PROGRAM MAIN
VAR
	bInitialized 		: 	BOOL := FALSE;
	bDeinitialize		:	BOOL;
	bCheck				:	BOOL;
	fbInit 				: 	FB_VN_InitializeFunction;	
	nReturnCode			:   UDINT;
	
	hr					:	HRESULT;
	hrCheck				:	HRESULT;
	hrDeinitialize		:	HRESULT;
	hrOCR				:	HRESULT;
	fbCameraControl		:	FB_VN_FileSourceControl;
	eCameraState		:	ETcVnCameraState;
	sFileName 			: 	STRING;
	ImageCounter		:	UINT;

	stPixelFormat		:	TcVnPixelFormat;
	stRoi				:	TcVnRectangle_UDINT;
	fThreshold			:	LREAL;
	bInvertImage		:	BOOL := TRUE;
	
	ipOriginalImage		:	ITcVnImage; 
	ipBinaryImage		:	ITcVnImage; 
	ipThreshBorder		:	ITcVnImage;
	ipStructElem		: 	ITcvnImage;
	ipOriginImageDisp	:	ITcVnDisplayableImage;
	ipBinImageDisp		:	ITcVnDisplayableImage;
	ipThreshBorderDisp	:	ITcVnDisplayableImage;
	
	aRedColor			: 	TcVnVector4_LREAL := [255,0,0];
	aGreenColor			: 	TcVnVector4_LREAL := [0,255,0];
	aBlueColor			: 	TcVnVector4_LREAL := [0,0,255];
	aWhiteColor			: 	TcVnVector4_LREAL := [255,255,255];
	
	// OCR
	bUseExpFunction		:	BOOL := FALSE;
	ipOCRResult 		:	ITcVnContainer; (* Returns the detected characters (ContainerType_Vector_String_SINT) *)
	sText 				: 	STRING(255);
	nStringLenght		:	INT;

	// OCR Exp
	sPattern			:	STRING;			(* String template containing the format in which characters are presented *)
	eOcrOptions			:	UDINT;			(* Specifies which options must be applied to the function (ETcVnOcrOptions) *)
	ipBoundingBoxes		:	ITcVnContainer;	(* Returns the corresponding bounding boxes of the detected characters (ContainerType_Vector_TcVnRectangle_DINT, optional, set to 0 if not required) *)
	ipConfidences		:	ITcVnContainer;	(* Returns the corresponding classification confidences of the detected characters (ContainerType_Vector_REAL, optional, set to 0 if not required) *)
	fMinConfidence		:	REAL;			(* Returns the minimum value of the confidences *)
	
	nNumberOfElements	: 	ULINT;
	nIterator			: 	ULINT;
	aConfidences		:	ARRAY [0..11] OF REAL;
	stRectangle			:	TcVnRectangle_DINT;
END_VAR

// Disclaimer

// This publication contains statements about the suitability of our products for certain
// areas of application. These statements are based on typical features of our products.
// The examples shown in this publication are for demonstration purposes only.
// The information provided herein should not be regarded as specific operation characteristics.
// It is incumbent on the customer to check and decide whether a product is suitable for use
// in a particular application. We do not give any warranty that the source code which is
// made available with this publication is complete or accurate.

// THE SAMPLE CODE CONTAINED IN THIS PUBLICATION IS PROVIDED “AS IS” WITHOUT WARRANTY OF ANY KIND,
// EITHER EXPRESSED, IMPLIED OR STATUTORY, INCLUDING WITHOUT LIMITATION, ANY WARRANTY WITH RESPECT TO NON-INFRINGEMENT,
// FREEDOM FROM PROPRIETARY RIGHTS OF THIRD PARTIES OR FITNESS FOR ANY PARTICULAR PURPOSE.

// This publication may be changed from time to time without prior notice.
// No liability is assumed for errors and/or omissions.
// Our products are described in detail in our data sheets and documentations.
// Product-specific warnings and cautions must be observed.
// For the latest version of our data sheets and documentations visit our website (www.beckhoff.de).

// © Beckhoff Automation GmbH & Co. KG, December 2023

// The reproduction, distribution and utilization of this document as well as the communication
// of its contents to others without express authorization is prohibited. 
// Offenders will be held liable for the payment of damages.
// All rights reserved in the event of the grant of a patent, utility model or design.

//	==========================================================================================

// SAMPLE - OCR (Optical Character Recognition)
//	-------------------------------------------------------

// Steps To Do:
// ------------
// 1. Add the sample images to the FileSource1 Control
// 2. Activate the Configuration -> Start TwinCAT System and PLC to run -> watch the results in the ADS Image Watch
// 3. Switch between OCR standard and expert function with bUseExpFunction

// Load OCR Model
IF NOT bInitialized THEN
	fbInit(eFunction := TCVN_IF_OCR, nOptions := ETcVnOcrModelType.TCVN_OMT_NUMBERS_SC_UCLETTERS OR ETcVnOcrModelType.TCVN_OMT_NUMBERS_SC OR ETcVnOcrModelType.TCVN_OMT_UCLETTERS, bStart := TRUE);
	
	IF NOT fbInit.bBusy THEN
		fbInit(bStart := FALSE);
		IF NOT fbInit.bError THEN
			bInitialized := TRUE;
			nReturnCode := fbInit.nErrorId AND 16#FFF;
		ELSE
			nReturnCode := fbInit.nErrorId AND 16#FFF;
		END_IF
	END_IF
END_IF

// Check if Model is initialized
IF bCheck THEN
	bCheck := FALSE;
	hrCheck := F_VN_CheckFunctionInitialization(eFunction := TCVN_IF_OCR, nOptions := ETcVnOcrModelType.TCVN_OMT_NUMBERS_SC, hrPrev := S_OK);
END_IF

// Unload OCR Model
IF bDeinitialize THEN
	bDeinitialize := FALSE;
	hrDeinitialize := F_VN_DeinitializeFunction(eFunction:= TCVN_IF_OCR, nOptions:= ETcVnOcrModelType.TCVN_OMT_NUMBERS_SC, hrPrev:= S_OK);
	bInitialized := FALSE;
END_IF

// Get Camera State
eCameraState := fbCameraControl.GetState();
	
// CameraControl is in error state, so try to reset the camera connection
IF eCameraState = TCVN_CS_ERROR THEN
	hr := fbCameraControl.Reset();

// Camera not yet streaming
ELSIF eCameraState < TCVN_CS_ACQUIRING THEN
	hr := fbCameraControl.StartAcquisition();

// Camera streaming
ELSIF eCameraState = TCVN_CS_ACQUIRING THEN	
	
	hr := fbCameraControl.GetCurrentImageAndFileName(ipImage := ipOriginalImage, sFileName := sFileName, 80);
	
	IF bInitialized AND SUCCEEDED(hr) AND ipOriginalImage <> 0 THEN
		
		ImageCounter := ImageCounter + 1;
		
		// Check pixel format and prepare work image
		hr := F_VN_GetPixelFormat(ipOriginalImage, stPixelFormat, hr);			
		IF stPixelFormat.nChannels = 3 AND stPixelFormat.ePixelEncoding = TCVN_PE_NONE THEN
			hr := F_VN_ConvertColorSpace(ipOriginalImage, ipBinaryImage, TCVN_CST_RGB_TO_GRAY, hr);			
		ELSE
			hr := F_VN_CopyImage(ipOriginalImage, ipBinaryImage, hr);
		END_IF
		
		// Helper funtion to get ROI and threshold value according to sample image
		F_GetROI(sFileName, stRoi, fThreshold, bInvertImage, sPattern);
			 
		// Set ROI and draw rectangle
		hr := F_VN_SetRoi_TcVnRectangle_UDINT(stRoi, ipBinaryImage, hr);
		hr := F_VN_DrawRectangle_TcVnRectangle_UDINT(stRoi, ipOriginalImage, aRedColor, 2, hr);
		
		// Filter Image 
		// Add or replace pre-processing functions if needed
		hr := F_VN_CreateStructuringElement(ipStructElem, ETcVnStructuringElementShape.TCVN_SES_RECTANGLE, 3,3, hr);
		hr := F_VN_MorphologicalOperator(ipBinaryImage, ipBinaryImage, ETcvnMorphologicalOperator.TCVN_MO_CLOSING_BY_RECONSTRUCTION, ipStructElem, hr);	

////		// Invert image depending on bright or dark text color 
		IF bInvertImage THEN
			hr := F_VN_Threshold(ipBinaryImage, ipBinaryImage, fThreshold, 255, TCVN_TT_BINARY_INV, hr);
		ELSE
			hr := F_VN_Threshold(ipBinaryImage, ipBinaryImage, fThreshold, 255, TCVN_TT_BINARY, hr);
		END_IF
		
		// Remove border objects
		hr := F_VN_BrightBorderObjects(ipBinaryImage, ipThreshBorder, hr);
		hr := F_VN_SubtractImages(ipBinaryImage, ipThreshBorder, ipBinaryImage, hr);
	
		// Read characters
		IF NOT bUseExpFunction THEN
			hrOCR := F_VN_OCR(
					ipSrcImage		:= ipBinaryImage,
					eModel			:= ETcVnOcrModelType.TCVN_OMT_NUMBERS_SC_UCLETTERS,
					ipCharacters	:= ipOCRResult,
					hrPrev			:= hr);
			hrOCR := F_VN_OCR(
					ipSrcImage		:= ipBinaryImage,
					eModel			:= ETcVnOcrModelType.TCVN_OMT_NUMBERS,
					ipCharacters	:= ipOCRResult,
					hrPrev			:= hr);
		ELSE
			hrOCR := F_VN_OCRExp(
					ipSrcImage		:= ipBinaryImage,
					eModel			:= ETcVnOcrModelType.TCVN_OMT_NUMBERS_SC or ETcVnOcrModelType.TCVN_OMT_UCLETTERS,
					ipCharacters	:= ipOCRResult, 
					sPattern		:= sPattern,
					eOcrOptions		:= eOcrOptions,
					ipBoundingBoxes	:= ipBoundingBoxes, 
					ipConfidences	:= ipConfidences,
					hrPrev			:= hr,
					fMinConfidence	=> fMinConfidence);
		END_IF
				
		// Check if characters were found
		hr := F_VN_GetNumberOfElements(ipOCRResult, nNumberOfElements, hrOCR);
		IF SUCCEEDED(hr) AND nNumberOfElements > 0 THEN
			// Export character to string
			hr := F_VN_ExportSubContainer_String(ipOCRResult, 0, sText, 255, hr);
			nStringLenght := LEN(sText);
			
			// Write text result to filtered and original image
			hr := F_VN_PutText(sText, ipBinaryImage,  12, 12, TCVN_FT_HERSHEY_PLAIN, 1, aWhiteColor, hr);
			hr := F_VN_PutText(sText, ipOriginalImage, stRoi.nX + 5, stRoi.nY + 25, TCVN_FT_HERSHEY_DUPLEX, 1, aGreenColor, hr);
			
			IF bUseExpFunction THEN 
				// Get number of Confidence elements and export them if array is large enough 
				MEMSET(ADR(aConfidences), 0, SIZEOF(aConfidences));
				hr := F_VN_GetNumberOfElements(ipConfidences, nNumberOfElements, hr);
				
				// Check if number of elements fits to array size
				IF nNumberOfElements > 0 AND nNumberOfElements <= 12 THEN
					hr := F_VN_ExportContainer(ipConfidences, ADR(aConfidences), SIZEOF(aConfidences), hr);
				END_IF
				
				// Get bounding box rectangle and draw it to filtered and original image
				hr := F_VN_GetNumberOfElements(ipBoundingBoxes, nNumberOfElements, hr);
				IF nNumberOfElements > 0 THEN
					FOR nIterator := 0 TO nNumberOfElements -1 DO
						hr := F_VN_GetAt_TcVnRectangle_DINT(ipBoundingBoxes, stRectangle, nIterator, hr);
						hr := F_VN_DrawRectangle_TcVnRectangle_DINT(stRectangle, ipBinaryImage, aWhiteColor, 1, hr);
						// Add ROI Offset
						stRectangle.nX := stRectangle.nX + UDINT_TO_DINT(stRoi.nX);
						stRectangle.nY := stRectangle.nY + UDINT_TO_DINT(stRoi.nY);
						hr := F_VN_DrawRectangle_TcVnRectangle_DINT(stRectangle, ipOriginalImage, aBlueColor, 1, hr);
					END_FOR
				END_IF
			END_IF
		END_IF
		
		// Display images
		hr := F_VN_TransformIntoDisplayableImage(ipOriginalImage, ipOriginImageDisp, S_OK);
		hr := F_VN_TransformIntoDisplayableImage(ipBinaryImage, ipBinImageDisp, S_OK);
		hr := F_VN_TransformIntoDisplayableImage(ipThreshBorder, ipThreshBorderDisp, S_OK);
		 
		// Release Pointer
		hr := FW_SafeRelease(ADR(ipOCRResult));
		hr := FW_SafeRelease(ADR(ipBoundingBoxes));
		hr := FW_SafeRelease(ADR(ipConfidences));
	END_IF
END_IF

END_PROGRAM
